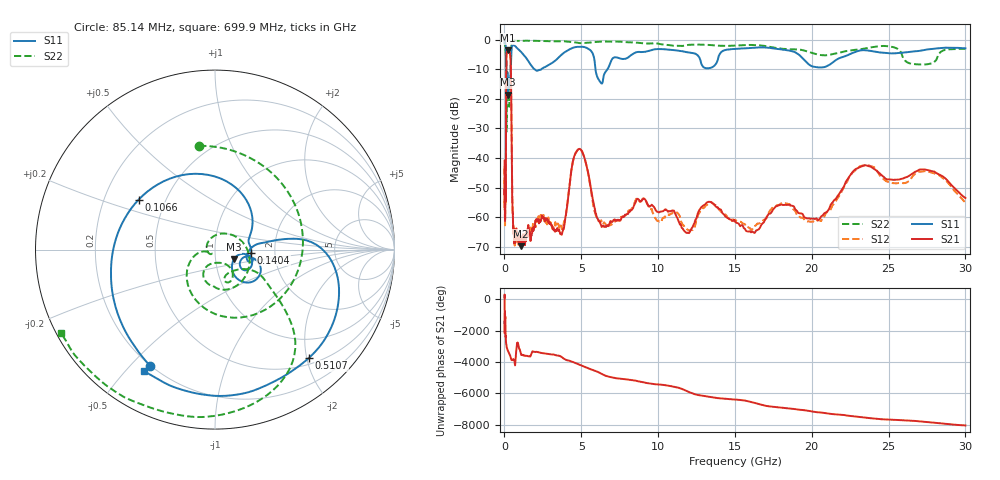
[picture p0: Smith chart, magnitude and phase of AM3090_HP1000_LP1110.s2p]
! Date/Time: Thu, Feb 28, 2019 2:02 PM
! Network Analyzer: Agilent Technologies E8364B Rev: A.07.50.67
! Sweep from 0.010 to 30.000 GHz, 1601 Points, Sweep Type: LOG
! Power Supply: 5.023 V, 0.002 A
# Hz S DB R 50
!freq MagS11 AngS11 MagS21 AngS21 MagS12 AngS12 MagS22 AngS22
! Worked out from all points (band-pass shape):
!   1601 points, 10 MHz to 30 GHz, reference 50 ohm
!   highest |S21| = -3.57 dB at 239.9 MHz (marker M1); lowest = -69.9 dB at 1.055 GHz (marker M2)
!   |S21| within 3 dB of the highest: 124.1 MHz to 399.1 MHz (275 MHz wide, 105 % of centre)
!   lowest |S11| = -18.6 dB at 241.1 MHz (marker M3), VSWR 1.27, Z = 61.3 - j6.79 ohm
!   |S11| at or under -10 dB: 118.4 MHz to 414.5 MHz (296.1 MHz wide, 111 % of centre); 1.971 GHz to 2.385 GHz (414.2 MHz wide, 19 % of centre); 5.925 GHz to 6.696 GHz (771.2 MHz wide, 12.2 % of centre)
!   |S22| runs from -31.1 to -0.2 dB; largest |S21 - S12| = 0.012
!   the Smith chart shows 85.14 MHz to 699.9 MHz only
!   S11 on the Smith chart (normalised r, x): 85.14 MHz: 0.20, -0.57; 106.6 MHz: 0.35, +0.26; 140.4 MHz: 1.51, -0.05; 510.7 MHz: 0.61, -2.04; 699.9 MHz: 0.16, -0.56
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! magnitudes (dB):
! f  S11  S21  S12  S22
! 10 MHz  -0.2  -40.9  -46.0  -0.7
! 38.04 MHz  -0.5  -60.4  -60.4  -1.6
! 85.14 MHz  -2.6  -53.2  -54.4  -4.7
! 106.6 MHz  -5.9  -22.6  -22.6  -6.7
! 140.4 MHz  -13.8  -4.5  -4.5  -27.7
! 144.7 MHz  -13.9  -4.3  -4.3  -26.6
! 239.9 MHz  -18.5  -3.6  -3.5  -13.9
! 241.1 MHz  -18.6  -3.6  -3.5  -13.9
! 309.6 MHz  -15.4  -3.8  -3.7  -22.6
! 405.7 MHz  -11.2  -7.3  -7.3  -8.9
! 510.7 MHz  -2.0  -54.7  -53.5  -0.5
! 550.5 MHz  -1.8  -60.1  -60.4  -0.4
! 699.9 MHz  -2.1  -66.8  -68.9  -0.2
! 1.055 GHz  -4.0  -69.9  -67.6  -0.3
! 2.084 GHz  -10.4  -60.9  -61.5  -0.3
! 3.742 GHz  -4.9  -65.8  -64.1  -0.4
! 4.854 GHz  -2.4  -36.9  -36.9  -1.1
! 6.234 GHz  -14.2  -62.1  -61.4  -0.6
! 7.926 GHz  -6.3  -59.1  -58.9  -0.8
! 16.21 GHz  -2.6  -65.2  -63.1  -1.7
! 23.48 GHz  -3.5  -42.4  -42.5  -2.9
! 30 GHz  -2.8  -53.5  -55.1  -3.0
